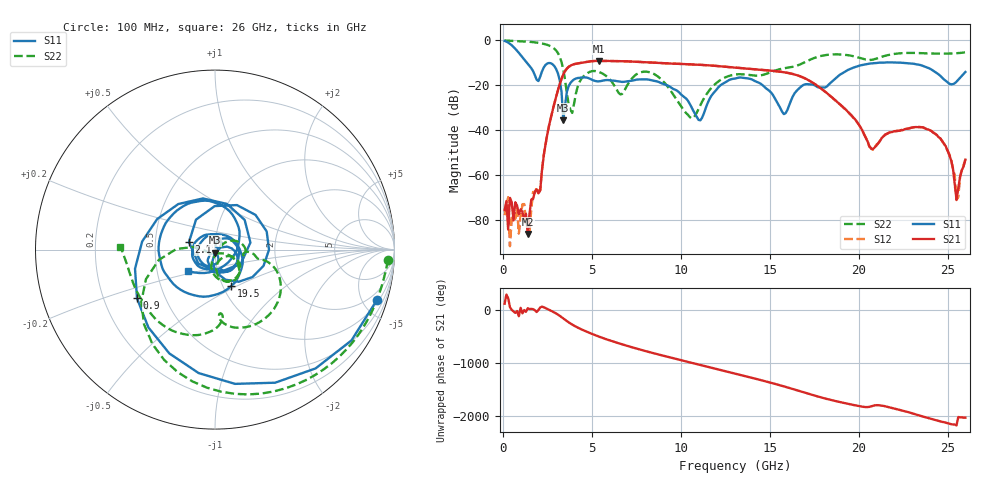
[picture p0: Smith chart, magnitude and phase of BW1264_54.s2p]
!Keysight Technologies,N5245B,MY57181159,A.13.60.06
!Date: Friday, December 18, 2020 23:54:55
!Correction: S11(Full 2 Port(1,2))
!S21(Full 2 Port(1,2))
!S12(Full 2 Port(1,2))
!S22(Full 2 Port(1,2))
!S2P File: Measurements: S11, S21, S12, S22:
# Hz S  dB  R 50
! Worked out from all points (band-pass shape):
!   260 points, 100 MHz to 26 GHz, reference 50 ohm
!   highest |S21| = -9.39 dB at 5.4 GHz (marker M1); lowest = -86.4 dB at 1.4 GHz (marker M2)
!   |S21| within 3 dB of the highest: 3.654 GHz to 13.06 GHz (9.406 GHz wide, 113 % of centre)
!   lowest |S11| = -35.8 dB at 3.4 GHz (marker M3), VSWR 1.03, Z = 49.9 - j1.62 ohm
!   |S11| at or under -10 dB: 1.328 GHz to end of sweep
!   |S22| runs from -34.9 to -0.3 dB; largest |S21 - S12| = 0.00055
!   S11 on the Smith chart (normalised r, x): 100 MHz: 1.21, -6.37; 900 MHz: 0.35, -0.25; 2.1 GHz: 0.74, +0.06; 19.5 GHz: 1.09, -0.47; 26 GHz: 0.72, -0.18
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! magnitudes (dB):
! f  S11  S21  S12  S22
! 100 MHz  -0.5  -75.8  -78.0  -0.3
! 900 MHz  -5.8  -77.6  -86.1  -0.6
! 1.4 GHz  -10.7  -86.4  -82.6  -0.8
! 2.1 GHz  -16.4  -67.0  -66.8  -1.5
! 3 GHz  -13.0  -25.2  -25.2  -4.8
! 3.4 GHz  -35.8  -15.4  -15.4  -13.3
! 3.9 GHz  -18.3  -11.1  -11.1  -32.5
! 4.5 GHz  -16.7  -10.2  -10.2  -16.5
! 5.4 GHz  -18.5  -9.4  -9.4  -14.3
! 6.6 GHz  -18.7  -9.5  -9.5  -24.2
! 8.8 GHz  -18.9  -10.4  -10.4  -16.9
! 10.6 GHz  -29.9  -10.9  -10.9  -34.9
! 13.1 GHz  -17.2  -12.4  -12.4  -15.4
! 15.8 GHz  -33.0  -14.4  -14.4  -12.7
! 17.4 GHz  -19.9  -19.0  -19.0  -8.4
! 19.5 GHz  -13.1  -32.9  -32.9  -7.0
! 20.8 GHz  -10.4  -48.7  -48.9  -8.8
! 21.7 GHz  -10.0  -41.3  -41.3  -6.7
! 24.6 GHz  -16.1  -43.9  -43.9  -6.2
! 25.2 GHz  -19.8  -53.6  -53.5  -6.1
! 25.5 GHz  -18.6  -71.1  -71.3  -6.0
! 26 GHz  -14.3  -53.3  -53.2  -5.6
